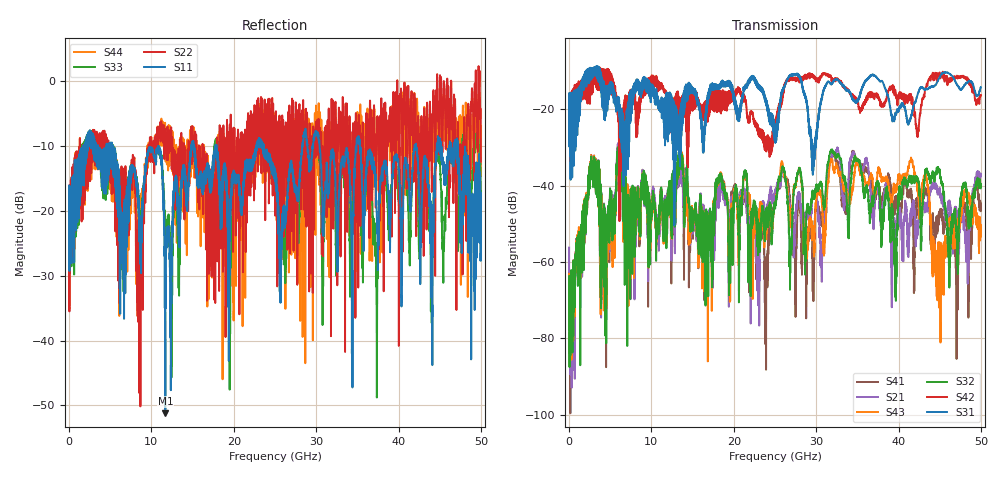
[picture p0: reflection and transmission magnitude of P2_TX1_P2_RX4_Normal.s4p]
!Keysight Technologies,N5225B,MY57041031,A.13.20.10
!Date: Friday, May 31, 2019 11:32:23
!Correction: S11(Full 4 Port(1,2,3,4))
!S12(Full 4 Port(1,2,3,4))
!S13(Full 4 Port(1,2,3,4))
!S14(Full 4 Port(1,2,3,4))
!S21(Full 4 Port(1,2,3,4))
!S22(Full 4 Port(1,2,3,4))
!S23(Full 4 Port(1,2,3,4))
!S24(Full 4 Port(1,2,3,4))
!S31(Full 4 Port(1,2,3,4))
!S32(Full 4 Port(1,2,3,4))
!S33(Full 4 Port(1,2,3,4))
!S34(Full 4 Port(1,2,3,4))
!S41(Full 4 Port(1,2,3,4))
!S42(Full 4 Port(1,2,3,4))
!S43(Full 4 Port(1,2,3,4))
!S44(Full 4 Port(1,2,3,4))
!S4P File: Measurements: <S11,S12,S13,S14>,
!<S21,S22,S23,S24>,
!<S31,S32,S33,S34>,
!<S41,S42,S43,S44>:
# Hz S  dB  R 50.0
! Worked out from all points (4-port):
!   5000 points, 10 MHz to 50 GHz, reference 50 ohm
!   strongest paths, dB at 10 MHz, 12.51 GHz, 25.01 GHz, 37.51 GHz, 50 GHz:
!     S31: -19.5, -17.3, -28.8, -12.1, -14.3
!     S42: -19.7, -27.5, -23.7, -16.5, -16.3
!     S32: -65.9, -53.8, -45.4, -39.8, -39.6
!     S43: -63.1, -53.5, -44.5, -36.1, -52.2
!     S21: -56.2, -53.3, -42.0, -40.5, -37.6
!     S41: -62.8, -52.3, -43.1, -39.8, -45.6
!   lowest |S11| = -51.2 dB at 11.69 GHz (marker M1), VSWR 1.01, Z = 49.8 - j0.179 ohm
!   |S11| at or under -10 dB: 5.36 GHz to 10.81 GHz (5.449 GHz wide, 67.4 % of centre); 17.89 GHz to 22.7 GHz (4.805 GHz wide, 23.7 % of centre); 35.31 GHz to 41.96 GHz (6.643 GHz wide, 17.2 % of centre)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
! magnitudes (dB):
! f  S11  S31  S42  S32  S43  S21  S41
! 10 MHz  -19.5  -19.5  -19.7  -65.9  -63.1  -56.2  -62.8
! 2.79 GHz  -10.0  -11.8  -15.8  -34.3  -33.8  -34.2  -33.7
! 8.46 GHz  -20.3  -13.2  -18.0  -43.6  -42.8  -43.3  -43.4
! 11.69 GHz  -51.2  -23.1  -15.3  -44.1  -44.7  -43.2  -43.8
! 41.51 GHz  -19.0  -21.9  -16.2  -37.7  -32.7  -46.1  -41.2
! 44.7 GHz  -10.3  -12.8  -12.3  -36.4  -61.1  -41.6  -52.6
! 50 GHz  -17.3  -14.3  -16.3  -39.6  -52.2  -37.6  -45.6
